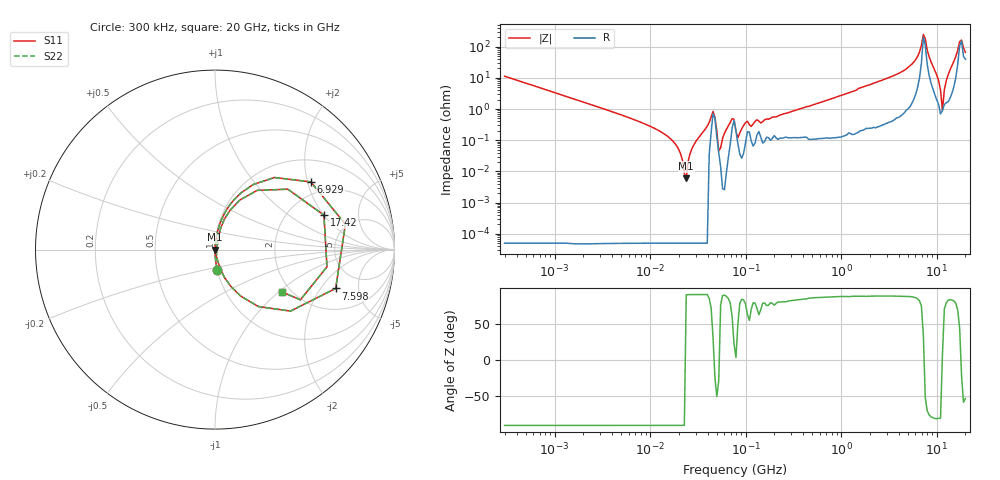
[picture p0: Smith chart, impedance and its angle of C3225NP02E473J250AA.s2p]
! S-parameter Generated by TDK Corporation
! Copyright(C) 2015 TDK Corporation.
! All Rights Reserved.
! TDK P/N: C3225NP02E473J250AA (Multilayer Ceramic Chip Capacitors)
! Property: C=47nF
! Size(LxWxT): 3.2x2.5x2.5mm, 0.126x0.098x0.098inches
! Model Type: s2p (Touchstone File Format Version 1.0)
! Frequency: DC=Yes Start=0.3MHz Stop=20000MHz 243points Log-sweep
! Note:
! Model Generated on Jun. 23, 2015
! Hash(MD5):
! Port Assignments:
!  1 ---| |--- 2
! Applicable Conditions:
!  Temperature = 25 degC
!  DC Bias Voltage = 0 V
!  Small Signal Operation
! Terms and conditions regarding TDK Simulation Models
! (1)This simulation model is being provided solely for informational purposes. Please refer to the specifications of the products in terms of detailed characteristics of such products.
! (2)In no event shall TDK Corporation of any of its subsidiaries be liable for any loss or damage arising, directly or indirectly,
!  From any information contained in this simulation model, including, but not limited to loss or damages arising from any inaccuracies, omissions or errors in connection with such information.
! (3)Any and all copyrights on this simulation model are owned by TDK Corporation.
!  Duplication or redistribution of this simulation model without prior written permission from TDK Corporation is prohibited.
! (4)This simulation model is subject to any modification or change without any prior notice.
! (5)Neither TDK Corporation nor any of its subsidiaries shall make any warranty, express or implied,
!  Including but not limited to the correctness, implied warranties of merchantability and fitness for a particular purpose with respect to this simulation models.
! (6)The use of this simulation model shall be deemed to have consented to the terms and conditions hereof.
# MHz S MA R 50
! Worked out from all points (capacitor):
!   242 points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, 300 kHz to 20 GHz, reference 50 ohm
!   read as one part in series: C = 46.9 nF near 314.2 kHz
!   lowest |Z| = 5.99 mohm at 23.91 MHz (marker M1)
!   series resonance near 23.48 MHz, so ESL is about 980 pH
!   S11 on the Smith chart (normalised r, x): 300 kHz: 1.00, -0.23; 6.929 GHz: 1.59, +2.10; 7.598 GHz: 3.25, -2.81; 17.42 GHz: 3.11, +2.01; 20 GHz: 1.79, -1.05
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0.3  0.1121 -83.6  0.9937 6.4  0.9937 6.4  0.1121 -83.6
1.985118  0.01692 -89.4  0.9998 1.0  0.9998 1.0  0.01692 -89.4
12.54397  0.001982 -94.9  0.9998 0.1  0.9998 0.1  0.001982 -94.9
23.91454  0.000178 160.3  0.9998 -0.0  0.9998 -0.0  0.000178 160.3
45.59205  0.008352 32.0  0.9929 -0.2  0.9929 -0.2  0.008352 32.0
47.74252  0.005544 -25.9  0.995 0.1  0.995 0.1  0.005544 -25.9
52.35254  0.0004463 -27.4  0.9996 0.0  0.9996 0.0  0.0004463 -27.4
72.28552  0.004915 59.7  0.9975 -0.2  0.9975 -0.2  0.004915 59.7
79.26541  0.001974 3.5  0.998 -0.0  0.998 -0.0  0.001974 3.5
83.00418  0.001202 49.5  0.9992 -0.1  0.9992 -0.1  0.001202 49.5
104.5156  0.004059 62.6  0.9981 -0.2  0.9981 -0.2  0.004059 62.6
500.8786  0.01342 84.7  0.9988 -0.8  0.9988 -0.8  0.01342 84.7
3165.055  0.1011 82.1  0.9912 -5.8  0.9912 -5.8  0.1011 82.1
5762.25  0.2996 69.0  0.9352 -17.4  0.9352 -17.4  0.2996 69.0
6928.783  0.6536 35.2  0.5982 -38.9  0.5982 -38.9  0.6536 35.2
7597.827  0.7063 -17.8  0.3902 32.9  0.3902 32.9  0.7063 -17.8
8724.45  0.2953 -61.2  0.8956 16.8  0.8956 16.8  0.2953 -61.2
10490.66  0.0808 -75.6  0.983 4.6  0.983 4.6  0.0808 -75.6
11503.64  0.008894 4.2  0.9911 -0.1  0.9911 -0.1  0.008894 4.2
12614.44  0.07974 74.2  0.9812 -4.5  0.9812 -4.5  0.07974 74.2
17417.32  0.6368 17.5  0.437 -26.0  0.437 -26.0  0.6368 17.5
20000  0.4401 -32.3  0.6709 20.5  0.6709 20.5  0.4401 -32.3
